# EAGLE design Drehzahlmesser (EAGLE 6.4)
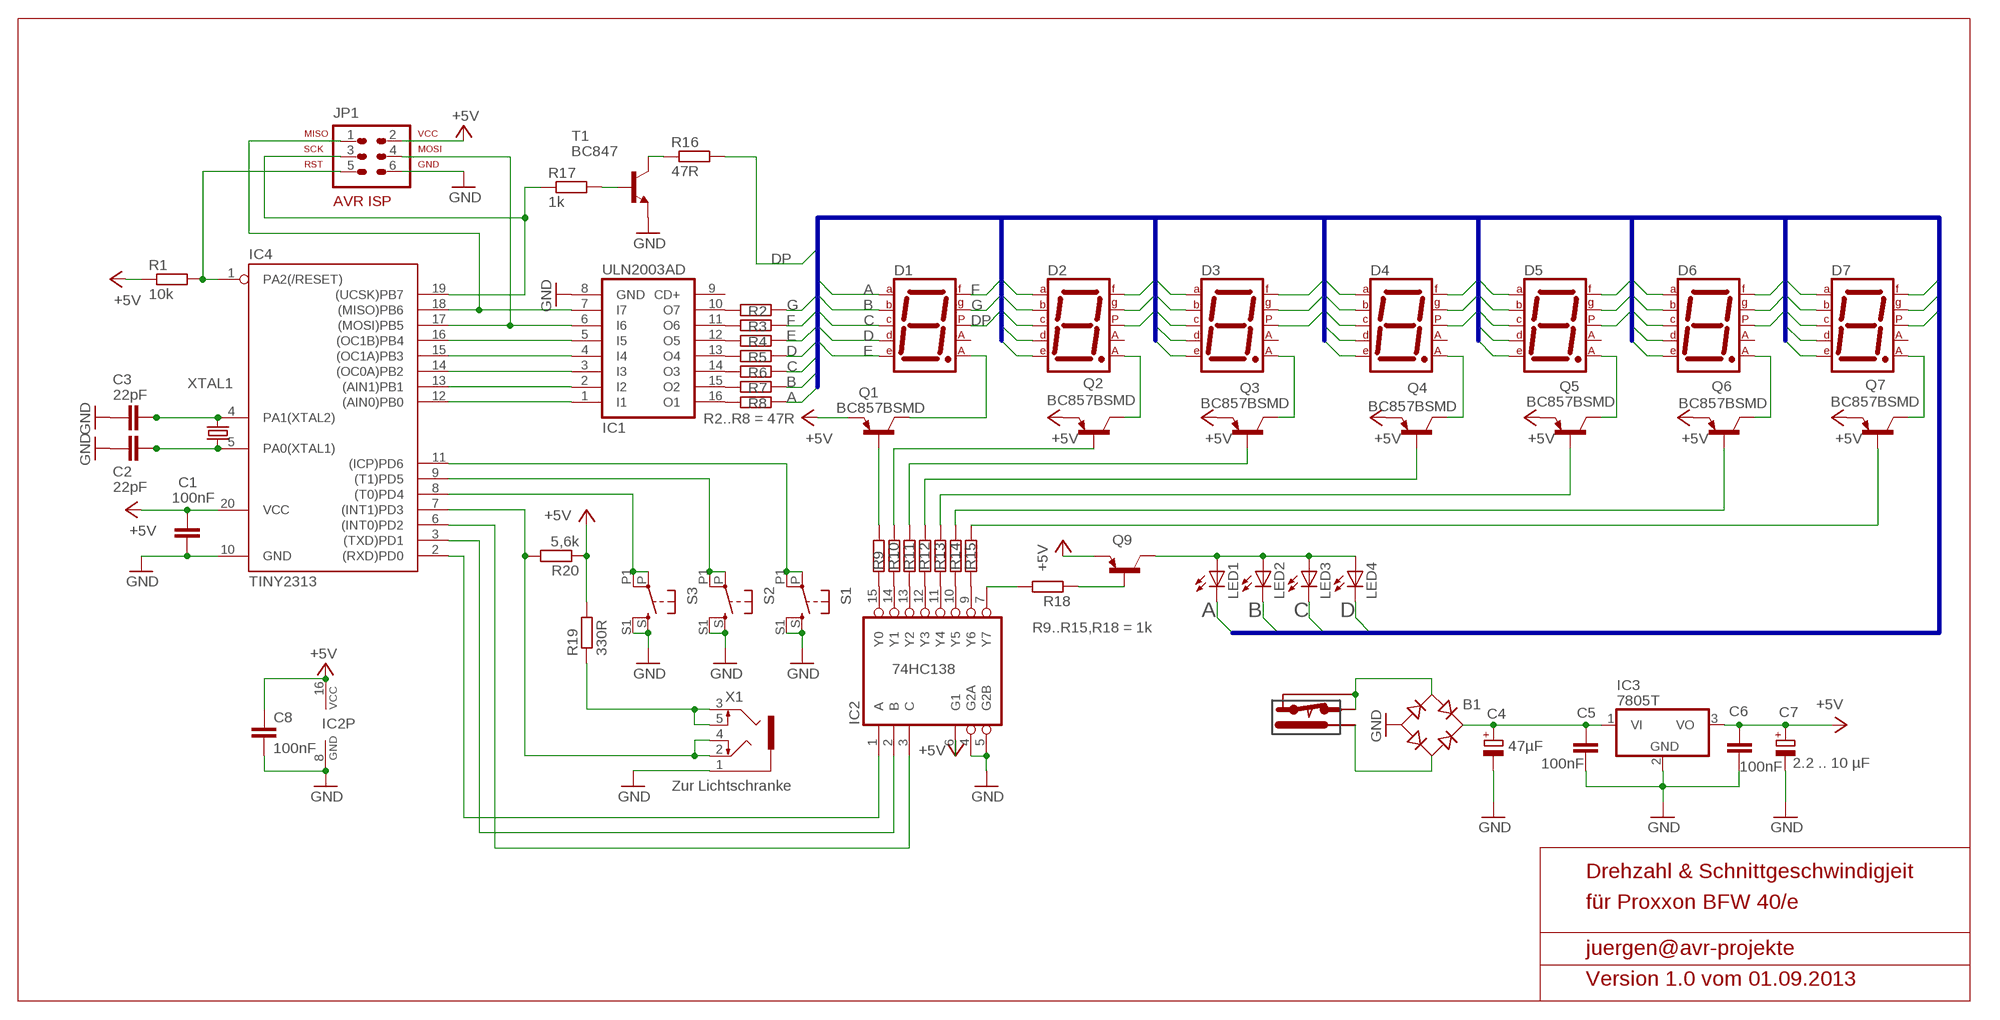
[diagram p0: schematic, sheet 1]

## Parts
B1  RECTIFIER-DIL  [B-DIL]
C1  100nF  C-EUC0805K  [C0805K]
C2  22pF  C-EUC0805  [C0805]
C3  22pF  C-EUC0805  [C0805]
C4  47µF  CPOL-EUE5-10.5  [E5-10,5]
C5  100nF  C-EUC0805K  [C0805K]
C6  100nF  C-EUC0805K  [C0805K]
C7  2.2 .. 10 µF  CPOL-EUE5-5  [E5-5]
C8  100nF  C-EUC0805K  [C0805K]
D1  7SEG-CA  [7SEG-13]
D2  7SEG-CA  [7SEG-13]
D3  7SEG-CA  [7SEG-13]
D4  7SEG-CA  [7SEG-13]
D5  7SEG-CA  [7SEG-13]
D6  7SEG-CA  [7SEG-13]
D7  7SEG-CA  [7SEG-13]
IC1  ULN2003AD  [SO16]
IC2  74HC138  74AC138D  [SO16]
IC3  7805T  [TO220H]
IC4  TINY2313  TINY2313-*S*  [SO20L$]
JP1  AVR-ISP-6VERT  [AVR-ISP-6]
LED1  LED3MM  [LED3MM]
LED2  LED3MM  [LED3MM]
LED3  LED3MM  [LED3MM]
LED4  LED3MM  [LED3MM]
Q1  BC857BSMD  [SOT23-BEC]
Q2  BC857BSMD  [SOT23-BEC]
Q3  BC857BSMD  [SOT23-BEC]
Q4  BC857BSMD  [SOT23-BEC]
Q5  BC857BSMD  [SOT23-BEC]
Q6  BC857BSMD  [SOT23-BEC]
Q7  BC857BSMD  [SOT23-BEC]
Q9  BC857BSMD  [SOT23-BEC]
R1  10k  R-EU_M0805  [M0805]
R2  R-EU_M0805  [M0805]
R3  R-EU_M0805  [M0805]
R4  R-EU_M0805  [M0805]
R5  R-EU_M0805  [M0805]
R6  R-EU_M0805  [M0805]
R7  R-EU_M0805  [M0805]
R8  R-EU_M0805  [M0805]
R9  R-EU_M0805  [M0805]
R10  R-EU_M0805  [M0805]
R11  R-EU_M0805  [M0805]
R12  R-EU_M0805  [M0805]
R13  R-EU_M0805  [M0805]
R14  R-EU_M0805  [M0805]
R15  R-EU_M0805  [M0805]
R16  47R  R-EU_M0805  [M0805]
R17  1k  R-EU_M0805  [M0805]
R18  R-EU_M0805  [M0805]
R19  330R  R-EU_M0805  [M0805]
R20  5,6k  R-EU_M0805  [M0805]
S1  TASTER-SMD-1612-11  [TASTER1612.11]
S2  TASTER-SMD-1612-11  [TASTER1612.11]
S3  TASTER-SMD-1612-11  [TASTER1612.11]
T1  BC847  [SOT23]
U$2  POWERBUCHSE21  [HEBW21]
X1  1503_09  [1503_09]
XTAL1  CRYSTALHC49S  [HC49/S]

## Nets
+5V: C1.1 C6.1 C7.+ C8.1 IC2.6(G1) IC2.16(VCC) IC3.3(VO) IC4.20(VCC) JP1.2 Q1.E Q2.E Q3.E Q4.E Q5.E Q6.E Q7.E Q9.E R1.1 R19.2 R20.1
A: D1.7(A) D2.7(A) D3.7(A) D4.7(A) D5.7(A) D6.7(A) D7.7(A) LED1.K(C) R8.2
B: D1.6(B) D2.6(B) D3.6(B) D4.6(B) D5.6(B) D6.6(B) D7.6(B) LED2.K(C) R7.2
C: D1.4(C) D2.4(C) D3.4(C) D4.4(C) D5.4(C) D6.4(C) D7.4(C) LED3.K(C) R6.2
D: D1.2(D) D2.2(D) D3.2(D) D4.2(D) D5.2(D) D6.2(D) D7.2(D) LED4.K(C) R5.2
DP: D1.5(DP) D2.5(DP) D3.5(DP) D4.5(DP) D5.5(DP) D6.5(DP) D7.5(DP) R16.2
E: D1.1(E) D2.1(E) D3.1(E) D4.1(E) D5.1(E) D6.1(E) D7.1(E) R4.2
F: D1.9(F) D2.9(F) D3.9(F) D4.9(F) D5.9(F) D6.9(F) D7.9(F) R3.2
G: D1.10(G) D2.10(G) D3.10(G) D4.10(G) D5.10(G) D6.10(G) D7.10(G) R2.2
GND: B1.- C1.2 C2.1 C3.1 C4.- C5.2 C6.2 C7.- C8.2 IC1.8(GND) IC2.4(G2A) IC2.5(G2B) IC2.8(GND) IC3.2(GND) IC4.10(GND) JP1.6 S1.S S1.S1 S2.S S2.S1 S3.S S3.S1 T1.2(E) X1.1
LS+: R19.1 X1.3 X1.5
LSOUT: IC4.7((INT1)PD3) R20.2 X1.2 X1.4
N$1: IC4.1(PA2(/RESET)) JP1.5 R1.2
N$2: IC1.1(I1) IC4.12((AIN0)PB0)
N$3: IC1.2(I2) IC4.13((AIN1)PB1)
N$4: IC1.3(I3) IC4.14((OC0A)PB2)
N$5: IC1.4(I4) IC4.15((OC1A)PB3)
N$6: IC1.5(I5) IC4.16((OC1B)PB4)
N$7: IC1.6(I6) IC4.17((MOSI)PB5) JP1.4
N$9: IC2.1(A) IC4.2((RXD)PD0)
N$10: IC2.2(B) IC4.3((TXD)PD1)
N$11: IC2.3(C) IC4.6((INT0)PD2)
N$12: IC1.10(O7) R2.1
N$13: IC1.11(O6) R3.1
N$14: IC1.12(O5) R4.1
N$15: IC1.13(O4) R5.1
N$16: IC1.14(O3) R6.1
N$17: IC1.15(O2) R7.1
N$18: IC1.16(O1) R8.1
N$19: IC2.15(Y0) R9.1
N$20: Q1.B R9.2
N$21: D1.8(CA2) Q1.C
N$22: D2.8(CA2) Q2.C
N$23: Q2.B R10.2
N$24: IC2.14(Y1) R10.1
N$25: IC2.13(Y2) R11.1
N$26: IC2.12(Y3) R12.1
N$27: IC2.11(Y4) R13.1
N$28: IC2.10(Y5) R14.1
N$29: IC2.9(Y6) R15.1
N$30: Q3.B R11.2
N$31: Q4.B R12.2
N$32: Q5.B R13.2
N$33: Q6.B R14.2
N$34: Q7.B R15.2
N$35: D3.8(CA2) Q3.C
N$36: D4.8(CA2) Q4.C
N$37: D5.8(CA2) Q5.C
N$38: D6.8(CA2) Q6.C
N$39: D7.8(CA2) Q7.C
N$40: IC4.19((UCSK)PB7) JP1.3 R17.1
N$41: R17.2 T1.1(B)
N$42: R16.1 T1.3(C)
N$43: C3.2 IC4.4(PA1(XTAL2)) XTAL1.2
N$44: C2.2 IC4.5(PA0(XTAL1)) XTAL1.1
N$46: IC4.11((ICP)PD6) S1.P S1.P1
N$47: IC4.9((T1)PD5) S2.P S2.P1
N$48: IC4.8((T0)PD4) S3.P S3.P1
N$49: IC2.7(Y7) R18.2
N$50: Q9.B R18.1
N$51: LED1.A LED2.A LED3.A LED4.A Q9.C
N$53: B1.AC2 U$2.STIFT
N$55: B1.+ C4.+ C5.1 IC3.1(VI)
N$56: B1.AC1 U$2.MASSE U$2.ÖFFNER
N$57: IC1.7(I7) IC4.18((MISO)PB6) JP1.1
Unconnected: D1.3(CA1) D2.3(CA1) D3.3(CA1) D4.3(CA1) D5.3(CA1) D6.3(CA1) D7.3(CA1) IC1.9(CD+)

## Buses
BUS:A,B,C,D,E,F,G,DP

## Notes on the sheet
- R2..R8 = 47R
- R9..R15,R18 = 1k
- Zur Lichtschranke
- Drehzahl & Schnittgeschwindigjeit
- für Proxxon BFW 40/e
- juergen@avr-projekte
- Version 1.0 vom 01.09.2013

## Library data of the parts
B1 = rectifier:RECTIFIER-: Rectifier
C1-C3 C5 C6 C8 = rcl:C-EU: CAPACITOR, European symbol
C4 C7 = rcl:CPOL-EU: POLARIZED CAPACITOR, European symbol
D1-D7 = special:7SEG-CA: 7-segment DISPLAY single anode, 13 mm
IC1 = uln-udn_x:ULN2003A: DRIVER ARRAY
IC2 = 74xx-eu:74*138: 3-line to 8-line DECODER/DEMULTIPLEXER
IC3 = linear:78*: Positive VOLTAGE REGULATOR Source: http://cache.national.com/ds/LM/LM78L05.pdf http://www.fairchildsemi.com/ds/LM/LM7805.pdf
IC4 = avr-7:TINY2313*: Atmel Tiny2313 2K Flash, 128 bytes EEPROM, 128 bytes RAM
JP1 = avr-7:AVR-ISP-6: AVR ISP-6 Serial Programming Header
LED1-LED4 = led:LED: LED
Q1-Q7 Q9 = transistor-pnp:BC857*: PNP Transistror
R1-R20 = rcl:R-EU_: RESISTOR, European symbol
S1-S3 = 0_jmw:TASTER-SMD-1612-11
T1 = transistor:BC847: NPN TRANSISTOR
U$2 = 0_jmw:POWERBUCHSE21
X1 = con-lumberg:1503_09: Jack connectors according to JISC 6560, 3.5 mm Klinkeneinbaukupplung nach JISC 6560, 3,5 mm, 3-polig/ stereo, abgewinkelte Ausführung, mit 2 Öffnern und Lötaugen, für Leiterplatten Rückseitenmontage Source: http://www.lumberg.com/Produkte/PDFs/1503_09.pdf; OC_FARNELL: 1243244; OC_NEWARK: unknown
XTAL1 = crystal:CRYSTAL: CRYSTAL; OC_FARNELL: 1667008; OC_NEWARK: unknown

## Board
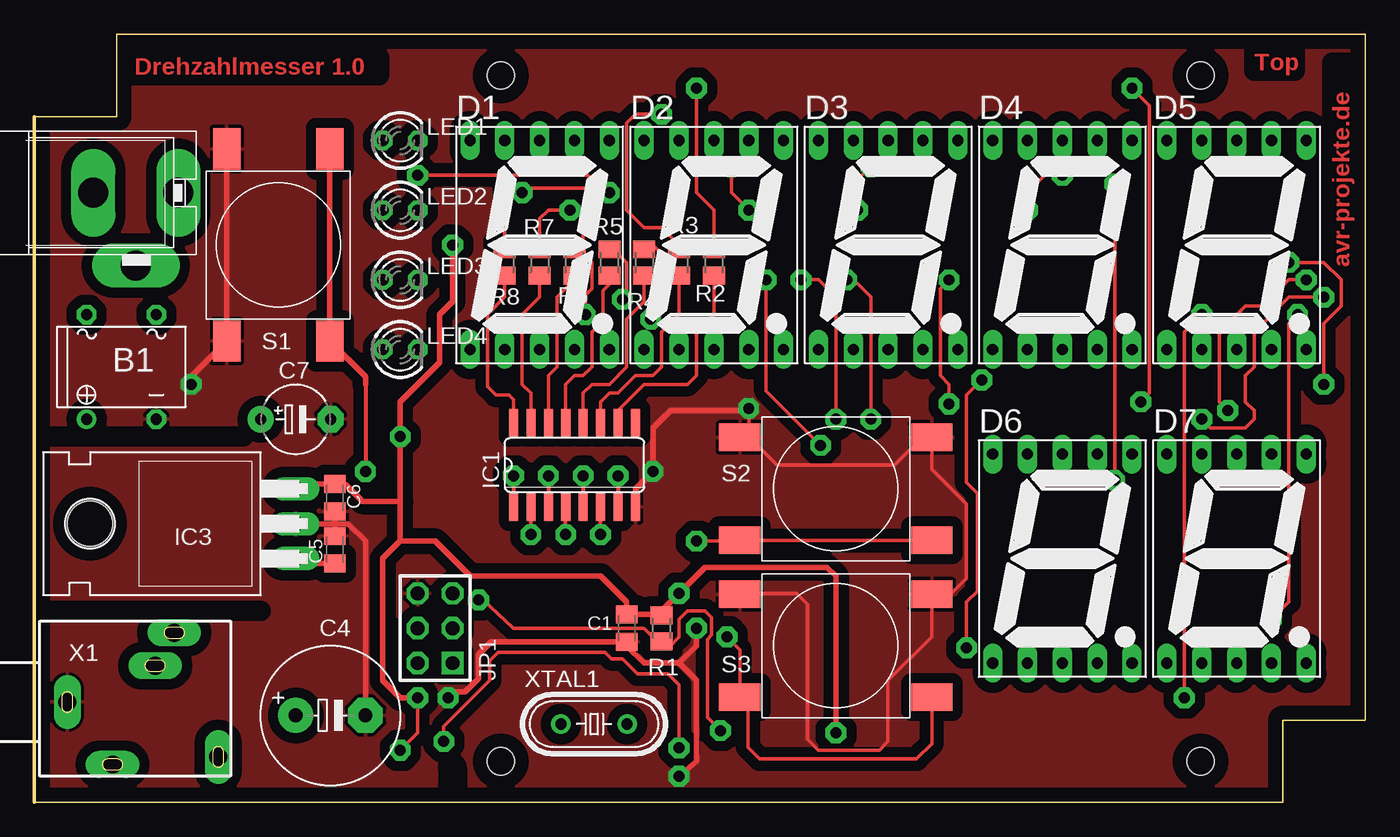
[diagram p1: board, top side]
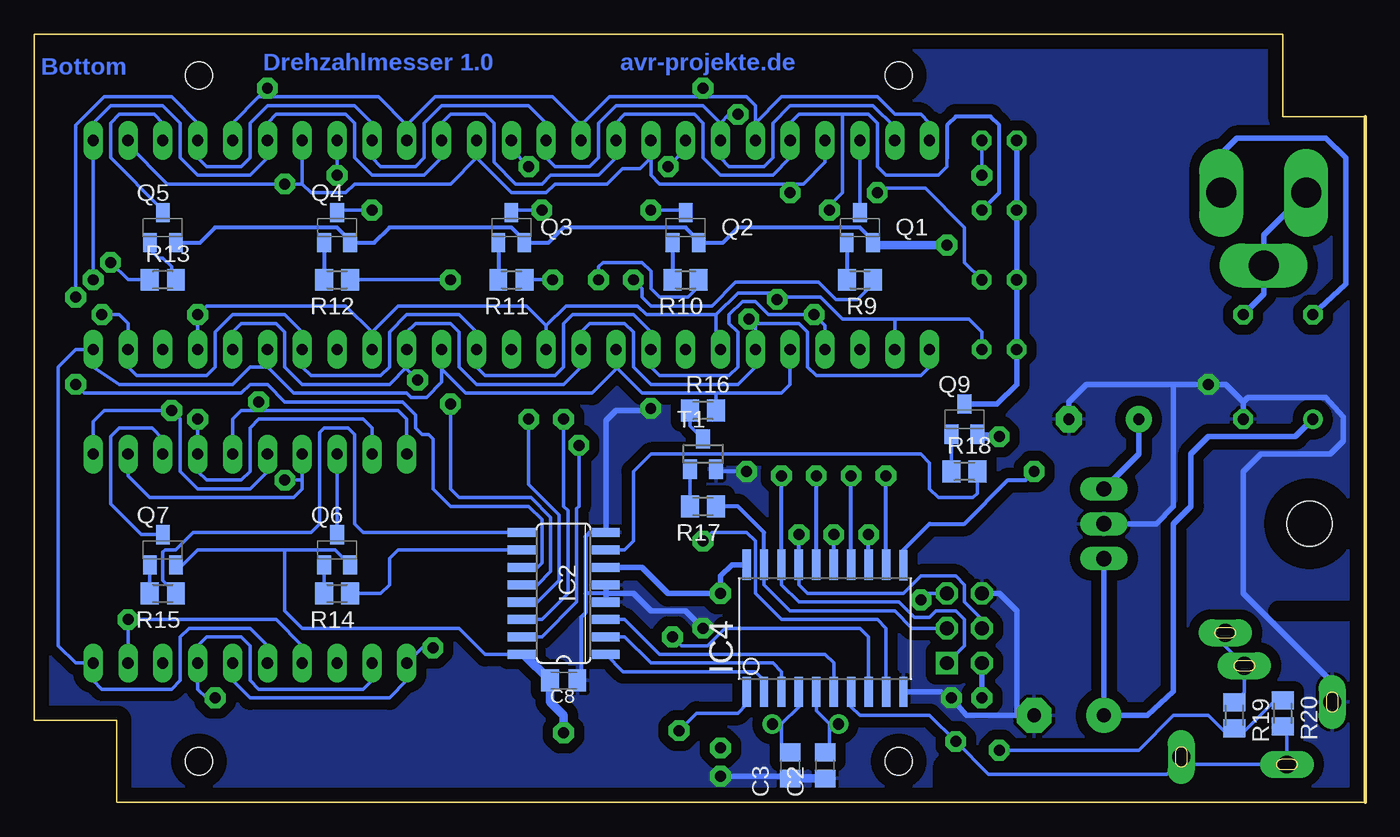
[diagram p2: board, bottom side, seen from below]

Size 97 x 56 mm. Coordinates in mm from the lower left corner, seen from the top.
Outline: 0,50 6,50 6,56 97,56 97,6 91,6 91,0 0,0 0,50
Copper layers (1*16): Top 0.035mm / dielectric 1.5mm / Bottom 0.035mm
Design rules "default *": minimum track width 10mil, minimum drill 24mil, track to track 8mil, track to pad 8mil, pad to pad 8mil, via to via 8mil, smd to smd 8mil, copper to edge 40mil, drill to drill 8mil, minimum pad ring 12mil, minimum via ring 14mil, stop-mask expansion 4mil, vias tented up to drill 0mil, thermal gap 10mil
Holes 2 mm at 34,53 85,53 85,3 34,3
tRestrict: 3 lines
bRestrict: 2 lines

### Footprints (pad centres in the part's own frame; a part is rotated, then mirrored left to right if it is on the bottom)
B-DIL = drill 0.813: + -2.54,-3.81 | drill 0.813 octagon: - 2.54,-3.81; AC1 2.54,3.81; AC2 -2.54,3.81
C0805K = smd 1.3 x 1.6: 1 -1,0; 2 1,0
C0805 = smd 1.3 x 1.5: 1 -0.95,0; 2 0.95,0
E5-10,5 = drill 1.016 pad 2.54: + -2.54,0 | drill 1.016 pad 2.54 octagon: - 2.54,0
E5-5 = drill 0.813 pad 1.905: + -2.54,0 | drill 0.813 pad 1.905 octagon: - 2.54,0
7SEG-13 = drill 0.813 long: 1 -5.08,-7.62; 2 -2.54,-7.62; 3 0,-7.62; 4 2.54,-7.62; 5 5.08,-7.62; 6 5.08,7.62; 7 2.54,7.62; 8 0,7.62; 9 -2.54,7.62; 10 -5.08,7.62
SO16 = smd 0.66 x 2.032: 1 -4.445,-3.073; 2 -3.175,-3.073; 3 -1.905,-3.073; 4 -0.635,-3.073; 5 0.635,-3.073; 6 1.905,-3.073; 7 3.175,-3.073; 8 4.445,-3.073; 9 4.445,3.073; 10 3.175,3.073; 11 1.905,3.073; 12 0.635,3.073; 13 -0.635,3.073; 14 -1.905,3.073; 15 -3.175,3.073; 16 -4.445,3.073
TO220H = drill 1.118 long: 1 -2.54,-10.16; 2 0,-10.16; 3 2.54,-10.16 | hole 3.302: 0,4.826
SO20L$ = smd 0.61 x 2.21: 1 -5.715,-4.636; 2 -4.445,-4.636; 3 -3.175,-4.636; 4 -1.905,-4.636; 5 -0.635,-4.636; 6 0.635,-4.636; 7 1.905,-4.636; 8 3.175,-4.636; 9 4.445,-4.636; 10 5.715,-4.636; 11 5.715,4.61; 12 4.445,4.636; 13 3.175,4.636; 14 1.905,4.636; 15 0.635,4.636; 16 -0.635,4.636; 17 -1.905,4.636; 18 -3.175,4.636; 19 -4.445,4.636; 20 -5.715,4.636
AVR-ISP-6 = drill 1.016 square: 1 -2.54,-1.27 | drill 1.016 octagon: 2 -2.54,1.27; 3 0,-1.27; 4 0,1.27; 5 2.54,-1.27; 6 2.54,1.27
LED3MM = drill 0.813 octagon: A -1.27,0; K 1.27,0
SOT23-BEC = smd 1 x 1.4: B -0.95,-1.1; C 0,1.1; E 0.95,-1.1
M0805 = smd 1.3 x 1.6: 1 -0.95,0; 2 0.95,0
TASTER1612.11 = smd 3 x 2: P -7,3.75; P1 7,3.75; S -7,-3.75; S1 7,-3.75
SOT23 = smd 1 x 1.4: 1 -0.95,-1.1; 2 0.95,-1.1; 3 0,1.1
HEBW21 = drill 2.184 pad 2.54 long: MASSE 0,6.5; STIFT 0,0.3; ÖFFNER -5.3,3.4
1503_09 = drill 1.3 pad 1.676 long: 1 0,-2.1; 2 -4.55,-5.4; 3 5.05,-9.9; 4 -4,-13.1; 5 2.65,-8.5
HC49/S = drill 0.813: 1 -2.413,0; 2 2.413,0

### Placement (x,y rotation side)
B1  6.35,31.75 0 top
C1  43.18,12.7 270 top
C2  39.37,2.7 90 bottom
C3  41.91,2.7 90 bottom
C4  21.59,6.35 0 top
C5  21.91,18.41 90 top
C6  21.91,22.23 270 top
C7  19.05,27.94 0 top
C8  58.42,8.89 0 bottom
D1  36.83,40.64 0 top
D2  49.53,40.64 0 top
D3  62.23,40.64 0 top
D4  74.93,40.64 0 top
D5  87.63,40.64 0 top
D6  74.93,17.78 0 top
D7  87.63,17.78 0 top
IC1  39.37,24.61 0 top
IC2  58.42,15.24 90 bottom
IC3  8.89,20.32 90 top
IC4  39.37,12.7 0 bottom
JP1  29.21,12.7 90 top
LED1  26.67,48.26 0 top
LED2  26.67,43.18 0 top
LED3  26.67,38.1 0 top
LED4  26.67,33.02 0 top
Q1  36.83,41.91 0 bottom
Q2  49.53,41.91 0 bottom
Q3  62.23,41.91 0 bottom
Q4  74.93,41.91 0 bottom
Q5  87.63,41.91 0 bottom
Q6  74.93,18.41 0 bottom
Q7  87.63,18.41 0 bottom
Q9  29.21,27.94 0 bottom
R1  45.72,12.7 270 top
R2  49.53,39.37 90 top
R3  46.99,39.37 90 top
R4  44.45,39.37 90 top
R5  41.91,39.37 90 top
R6  39.37,39.37 90 top
R7  36.83,39.37 90 top
R8  34.29,39.37 90 top
R9  36.83,38.1 180 bottom
R10  49.53,38.1 180 bottom
R11  62.23,38.1 180 bottom
R12  74.93,38.1 180 bottom
R13  87.63,38.1 0 bottom
R14  74.93,15.24 180 bottom
R15  87.63,15.24 180 bottom
R16  48.26,28.57 0 bottom
R17  48.26,21.59 180 bottom
R18  29.21,24.13 0 bottom
R19  9.53,6.35 270 bottom
R20  6,6.5 270 bottom
S1  17.78,40.64 270 top
S2  58.42,22.86 180 top
S3  58.42,11.43 180 top
T1  48.26,25.4 0 bottom
U$2  10.79,44.45 90 top
X1  0.3,7.32 90 top
XTAL1  40.8,5.71 0 top

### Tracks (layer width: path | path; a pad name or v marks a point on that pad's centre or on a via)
+5V  (via drill 0.8, 0.8 pad 0.81)
  Top 0.254: v26.67,3.81 27.94,5.08 v27.94,7.62
  Top 0.406: 45.67,13.7 C1.1 43.18,14.61 41.27,16.51 31.75,16.51 29.21,19.05 26.67,19.05 | 45.72,13.97 v46.99,15.24 48.9,17.14 57.78,17.14 58.42,16.51 v58.42,5.08 | 26.67,19.05 25.4,17.78 25.4,8.89 26.67,7.62 v27.94,7.62 | v30.48,40.64 30.48,36.51 29.53,35.56 29.53,32.07 26.67,29.21 v26.67,26.67 26.67,21.91 | 26.67,19.05 26.67,21.91 | 26.67,21.91 26.62,21.95 23.92,21.95 22.7,23.18 C6.1 19.41,23.23 IC3.3
  Top 0.61: 45.67,13.7 R1.1 45.72,13.97
  Bottom 0.254: Q7.E 86.19,17.32 85.09,18.41 78.74,18.41 | 78.74,18.41 75.08,18.41 Q6.E | IC2.16 64.14,10.79 66.04,12.7 77.47,12.7 78.74,13.97 78.74,18.41 | v26.67,3.81 16.51,3.81 13.97,6.35 11.43,6.35 10.16,5.08 | 9.85,5.08 8.92,5.08 6.5,7.5 6.05,7.5 R20.1
  Bottom 0.305: Q1.E 35.88,40.96 36.83,41.91 45.72,41.91 46.82,40.81 Q2.E 48.58,40.96 49.53,41.91 58.42,41.91 59.52,40.81 Q3.E 61.28,40.96 62.23,41.91 71.12,41.91 72.22,40.81 Q4.E 73.98,40.96 74.93,41.91 83.82,41.91 84.92,40.81 Q5.E
  Bottom 0.406: IC4.20 46.16,17.34 46.99,16.51 v46.99,15.24 50.8,15.24 52.7,17.14 IC2.6 | v27.94,7.62 JP1.2 | 10.16,5.08 9.85,5.08 R19.2 | C7.+ 16.51,25.4 IC3.3
  Bottom 0.61: v58.42,5.08 58.42,6.35 59.42,7.35 C8.1 61.33,10.79 IC2.16 | v26.67,26.67 28.09,26.67 Q9.E | v30.48,40.64 35.71,40.64 Q1.E
A  (via drill 0.8)
  Top 0.254: R8.2 34.29,45.72 | v78.74,23.5 v78.74,45.09 | 34.29,45.72 40.32,45.72 41.59,44.45 v41.91,44.45 | 34.29,45.72 v27.94,45.72
  Bottom 0.254: D5.7 90.17,47.94 87.31,45.09 v78.74,45.09 77.47,45.09 | 77.47,23.5 77.47,22.86 78.11,22.23 88.58,22.23 90.17,23.81 D7.7 | D6.7 77.47,23.5 | 77.47,23.5 v78.74,23.5 | D1.7 39.37,46.67 40.96,45.09 41.91,45.09 | v27.94,45.72 LED1.K | D2.7 52.07,46.99 | 52.07,46.99 52.07,45.72 51.44,45.09 41.91,45.09 | 64.77,46.99 62.23,44.45 59.69,44.45 59.05,45.09 55.24,45.09 54.13,46.2 52.86,46.2 52.07,46.99 | D3.7 64.77,46.99 | 64.77,46.99 66.67,45.09 73.66,45.09 74.3,44.45 76.83,44.45 77.47,45.09 | 77.47,45.09 D4.7 | v41.91,44.45 41.91,45.09
B  (via drill 0.8, 0.8 pad 0.81)
  Top 0.254: v87,28.57 86.36,29.21 86.36,34.29 88.27,36.2 89.53,36.2 91.44,38.1 v92.71,38.1 | R7.2 36.83,42.55 37.47,43.18 v39.05,43.18
  Bottom 0.254: D6.6 80.01,24.13 81.28,22.86 85.09,22.86 86.36,24.13 86.36,27.94 v87,28.57 91.92,28.57 92.71,27.78 D7.6 | v92.71,38.1 D5.6 92.71,49.53 91.44,50.8 87.63,50.8 86.36,49.53 86.36,46.99 85.09,45.72 81.28,45.72 80.01,46.99 D4.6 80.01,49.53 79.38,50.16 74.3,50.16 73.66,49.53 73.66,46.99 72.39,45.72 68.58,45.72 67.31,46.99 D3.6 67.31,49.53 66.67,50.16 64.14,50.16 63.5,49.53 63.5,46.67 61.91,45.09 60.01,45.09 59.37,45.72 55.88,45.72 54.61,46.99 D2.6 54.61,49.53 53.98,50.16 48.9,50.16 48.26,49.53 48.26,46.99 46.99,45.72 43.18,45.72 41.91,46.99 D1.6 41.91,49.53 41.27,50.16 38.1,50.16 | 38.1,50.16 36.2,50.16 35.56,49.53 35.56,46.35 34.92,45.72 31.11,45.72 30.48,46.35 30.48,46.99 30.48,47.62 | v39.05,43.18 39.05,43.5 38.1,44.45 38.1,50.16
  Bottom 0.305: LED2.K 26.67,44.45 26.67,49.37 27.3,50.01 29.84,50.01 30.48,49.37 30.48,46.99
C  (via drill 0.8, 0.8 pad 0.81)
  Top 0.254: v90.17,13.34 91.44,14.61 91.44,34.92 v92.08,35.56 | R6.2 39.05,40.32 | R6.2 39.69,40.32 40.64,39.37 40.64,37.47 40.16,36.99 v40.16,35.56 | v35.56,44.45 35.56,44.77 40.16,44.77 40.64,44.29 40.64,42.23 40.01,41.59 40.01,40.95 R6.2
  Bottom 0.254: D1.4 39.37,34.77 v40.16,35.56 43.5,35.56 44.45,36.51 45.4,36.51 46.35,35.56 46.35,34.92 45.72,34.29 45.72,31.75 46.35,31.11 51.44,31.11 52.07,31.75 D2.4 52.07,34.29 53.34,35.56 57.78,35.56 58.42,34.92 58.42,31.75 59.05,31.11 64.14,31.11 64.77,31.75 D3.4 64.77,34.29 66.04,35.56 69.85,35.56 71.12,34.29 71.12,31.75 71.75,31.11 76.83,31.11 77.47,31.75 D4.4 77.47,34.29 78.74,35.56 82.55,35.56 83.82,34.29 83.82,31.75 84.45,31.11 89.53,31.11 90.17,31.75 D5.4 90.17,34.92 90.81,35.56 v92.08,35.56 | D6.4 77.47,11.43 79.38,13.34 v90.17,13.34 D7.4 90.17,11.43 | LED3.K 29.21,39.37 29.21,41.91 32.07,44.77 35.56,44.77 v35.56,44.45
D  (via drill 0.8 pad 0.81)
  Top 0.254: v85.09,35.56 83.82,34.29 v83.82,7.62 | 41.59,40.32 R5.2 42.23,40.32 43.18,39.37 43.18,36.99 v42.86,36.67
  Bottom 0.254: D6.2 72.39,8.89 73.03,8.26 80.64,8.26 81.28,8.89 81.28,11.43 81.92,12.06 84.45,12.06 85.09,11.43 D7.2 85.09,8.26 84.45,7.62 v83.82,7.62 | D5.2 v85.09,35.56 84.45,36.2 74.3,36.2 72.39,34.29 | 47.31,35.56 52.39,35.56 53.02,36.2 58.26,36.2 59.69,34.77 | D2.2 46.99,33.66 47.31,33.97 47.31,35.56 | 47.31,35.56 45.72,37.15 43.34,37.15 v42.86,36.67 42.7,36.83 39.69,36.83 38.1,35.24 34.29,35.24 | 34.29,35.24 28.89,35.24 27.94,34.29 LED4.K | D1.2 34.29,35.24 | 59.69,34.77 61.12,36.2 70.48,36.2 72.39,34.29 | 72.39,34.29 D4.2 | 59.69,34.77 D3.2
DP
  Bottom 0.254: D6.5 80.01,11.43 81.28,12.7 85.72,12.7 86.36,12.06 86.36,8.89 87,8.26 92.08,8.26 92.71,8.89 D7.5 93.98,10.16 95.25,11.43 95.25,31.75 93.98,33.02 D5.5 92.71,31.75 90.81,30.48 82.55,30.48 81.28,31.75 80.01,31.75 | 41.91,31.75 D1.5 41.91,30.48 42.55,29.84 47.31,29.84 | 80.01,31.75 78.11,29.84 69.85,29.84 69.53,29.53 68.42,29.53 67.31,30.64 67.31,31.59 | 80.01,31.75 D4.5 | 46.99,29.21 46.99,28.57 R16.2 47.31,29.84 | 47.31,29.84 52.7,29.84 54.61,31.75 D2.5 54.61,31.59 56.36,29.84 65.56,29.84 67.31,31.59 | 67.31,31.59 D3.5
E  (via drill 0.8 pad 0.41, 0.8 pad 0.81)
  Top 0.254: 44.13,40.32 R4.2 44.77,40.64 45.09,40.64 45.72,40.01 45.72,36.04 v44.93,35.24 | v67.94,11.27 67.94,14.61 68.74,15.4 68.74,22.54 67.94,23.34 67.94,29.69 v69.06,30.8
  Bottom 0.254: D6.1 69.85,8.89 71.12,7.62 81.28,7.62 82.55,8.89 D7.1 | D1.1 31.75,31.75 32.38,31.11 40.01,31.11 40.64,31.75 40.64,34.29 41.27,34.92 44.45,34.92 | 44.45,34.92 D2.1 44.45,31.75 45.72,30.48 52.07,30.48 53.34,31.75 53.34,34.29 53.98,34.92 56.52,34.92 57.15,34.29 D3.1 57.15,31.75 58.42,30.48 64.77,30.48 66.04,31.75 66.04,34.29 66.67,34.92 69.22,34.92 69.85,34.29 D4.1 69.85,31.75 | 69.85,31.75 71.12,30.48 77.47,30.48 78.74,31.75 78.74,34.29 79.38,34.92 81.92,34.92 82.55,34.29 D5.1 | 44.45,34.92 v44.93,35.24 | D6.1 69.85,11.43 | v67.94,11.27 68.74,11.27 D6.1 | 69.85,31.75 69.85,31.59 v69.06,30.8
F  (via drill 0.8 pad 0.81)
  Top 0.254: v85.09,27.94 85.72,27.3 88.27,27.3 88.9,27.94 88.9,28.57 88.27,29.21 88.27,31.11 88.9,31.75 88.9,34.29 91.44,36.83 v93.98,36.83 | R3.2 46.99,40.64 45.72,41.91 44.45,41.91 43.18,43.18 43.18,49.53 43.81,50.16 v45.72,50.16
  Bottom 0.254: D1.9 34.29,49.21 35.88,50.8 41.91,50.8 43.18,49.53 43.18,46.99 43.81,46.35 46.35,46.35 46.99,46.99 D2.9 46.99,49.53 | 46.99,49.53 48.26,50.8 54.61,50.8 55.88,49.53 55.88,46.99 56.52,46.35 59.05,46.35 59.69,46.99 D3.9 59.69,49.53 60.96,50.8 67.31,50.8 68.58,49.53 68.58,46.99 69.22,46.35 71.75,46.35 72.39,46.99 D4.9 72.39,49.53 73.66,50.8 80.01,50.8 81.28,49.53 81.28,46.99 81.92,46.35 84.45,46.35 85.09,46.99 D5.9 85.09,49.53 87,51.44 91.92,51.44 93.98,49.37 v93.98,36.83 | D6.9 72.39,27.3 73.03,27.94 80.64,27.94 81.28,27.3 81.28,24.13 81.92,23.5 84.45,23.5 85.09,24.13 D7.9 v85.09,27.94 | v45.72,50.16 46.35,50.16 46.99,49.53
G  (via drill 0.8 pad 0.81)
  Top 0.254: v80.64,29.21 81.28,29.84 81.28,50.8 v80.01,52.07 | R2.2 49.53,43.18 48.26,44.45 v48.26,52.07
  Bottom 0.254: D1.10 31.75,49.53 32.38,50.16 34.29,50.16 35.56,51.44 42.55,51.44 44.45,49.53 | 80.01,51.44 80.64,51.44 82.55,49.53 D5.10 | D6.10 69.85,27.94 70.48,28.57 80.64,28.57 | 80.64,28.57 81.92,28.57 82.55,27.94 D7.10 | v80.64,29.21 80.64,28.57 | v48.26,52.07 48.26,51.44 | v80.01,52.07 80.01,51.44 | 44.45,49.53 D2.10 | 48.26,51.44 45.09,51.44 44.45,50.8 44.45,49.53 | 57.15,49.37 55.09,51.44 48.26,51.44 | D3.10 57.15,49.37 | 57.15,49.37 59.21,51.44 67.79,51.44 69.85,49.37 | 69.85,49.37 D4.10 | 80.01,51.44 71.91,51.44 69.85,49.37
GND  (via drill 0.8, 0.8 pad 0.81)
  Top 0.254: v52.07,28.73 52.07,27.26 51.77,26.96 | 51.77,26.96 S2.S1 | 50.74,15.18 S3.S1 51.48,15.24 55.56,15.24 56.36,14.45 56.36,4.6 57.15,3.81 61.59,3.81 62.23,4.45 62.23,8.89 65.42,12.08 S3.S 65.48,15.24 66.83,15.24 67.94,16.35 67.94,21.75 65.42,24.27 S2.S 65.36,26.67 64.77,26.67 62.71,24.61 54.13,24.61 51.77,26.96
  Top 0.406: C1.2 33.29,11.7 32.38,10.79 32.38,9.05 31.4,8.06 30.61,8.06 v30.16,7.62 | 43.18,11.43 44.45,10.16 46.99,10.16 | 46.99,10.16 48.26,11.43 v48.26,12.7 | 46.99,10.16 48.26,8.89 48.26,3.02 v46.99,1.91 | 52.07,28.57 46.35,28.57 45.09,27.3 v45.09,24.13 43.81,22.86 IC1.8 | C4.- 24.13,19.05 22.86,20.32 21.91,20.32 | C5.2 21.91,20.32 | 21.91,20.32 C6.2 | IC3.2 21.91,20.32 | v11.43,30.48 11.43,31.04 S1.S1 S1.S
  Top 0.61: C1.2 43.18,11.43
  Bottom 0.305: v45.09,24.13 47.14,24.13 T1.2 | IC2.8 56.52,19.68 56.83,19.37 56.83,15.24 | 56.83,15.24 56.83,13.81 57.15,13.49 57.15,9.48 | 55.35,15.24 56.83,15.24
  Bottom 0.406: IC2.4 55.35,15.24 | 55.35,15.24 IC2.5 55.35,15.34 55.24,15.24 | 55.24,15.24 53.34,15.24 52.07,13.97 49.53,13.97 v48.26,12.7 | 55.24,15.24 55.35,15.24 | C8.2 57.15,8.89 56.99,9.05 | v46.99,1.91 42.55,1.91 42.23,1.59 42.23,1.58 42.23,1.27 | IC2.8 55.35,27.84 54.61,28.57 52.07,28.57 | JP1.6 26.67,15.24 25.4,13.97 25.4,6.35 | C4.- 25.4,6.35 | 25.4,6.35 29.05,6.35 v30.16,7.62 30.92,8.06 IC4.10 | B1.- 8.89,29.21 | 8.89,29.21 10.16,30.48 v11.43,30.48 13.97,30.48 | 13.97,30.48 20.32,30.48 21.59,29.21 C7.- | 57.1,9.21 C8.2 | C8.2 56.99,9.32 57.15,9.48 | 8.89,29.21 8.57,29.53 2.86,29.53 1.59,28.1 1.59,26.35 2.54,25.4 7.62,25.4 8.89,24.13 8.89,15.24 2.4,8.75 X1.1 | 13.97,30.48 13.97,21.59 15.24,20.32 IC3.2
  Bottom 0.61: C3.1 C2.1
  pour Bottom (isolate 0.75): -1.27,-1.27 97.79,-1.27 97.79,57.15 -1.27,57.15
  pour Top (isolate 0.75): -1.27,57.15 -1.27,-1.27 97.79,-1.27 97.79,57.15
LS+
  Bottom 0.254: X1.3 10.2,11.37 X1.5 8.8,8.02 R19.1
LSOUT  (via drill 0.8)
  Top 0.254: v29.84,4.45 29.84,5.56 33.18,8.89 33.18,10.32 33.81,10.95 41.59,10.95 42.07,10.48 42.86,10.48 43.97,9.37 46.2,9.37 46.99,8.57 v46.99,3.97
  Bottom 0.254: IC4.7 37.47,6.99 36.83,6.35 31.75,6.35 v29.84,4.45 27.45,2.05 27.44,2.06 14.45,2.06 13.4,3.11 X1.4 12.85,2.77 X1.2 5.7,5.55 R20.2
N$1  (via drill 0.8 pad 0.81)
  Top 0.254: v32.38,14.76 32.7,14.76 34.92,12.7 44.45,12.7 45.4,11.75 R1.2 46.04,11.43 46.35,11.43 46.99,12.06 46.99,13.34 47.62,13.97 48.9,13.97 49.37,13.49 49.37,12.22 49.05,11.91 49.05,6.19 v50.01,5.24
  Bottom 0.254: v50.01,5.24 48.74,6.51 45.72,6.51 45.09,7.14 45.05,7.14 IC4.1 | v32.38,14.76 31.91,15.24 JP1.5
N$2  (via drill 0.8 pad 0.81)
  Top 0.305: v34.92,23.81 IC1.1
  Bottom 0.305: IC4.12 v34.92,23.81
N$3  (via drill 0.8 pad 0.81)
  Top 0.305: v36.2,19.53 IC1.2
  Bottom 0.305: IC4.13 v36.2,19.53
N$4  (via drill 0.8 pad 0.81)
  Top 0.305: v37.47,23.81 IC1.3
  Bottom 0.305: IC4.14 v37.47,23.81
N$5  (via drill 0.8 pad 0.81)
  Top 0.305: v38.73,19.53 IC1.4
  Bottom 0.305: IC4.15 v38.73,19.53
N$6  (via drill 0.8 pad 0.81)
  Top 0.305: v40.01,23.81 IC1.5
  Bottom 0.305: IC4.16 v40.01,23.81
N$7  (via drill 0.8 pad 0.81)
  Top 0.305: v41.27,19.53 IC1.6
  Bottom 0.254: JP1.4 27.94,13.34 29.21,14.61 29.21,15.88 29.84,16.51 32.38,16.51 33.66,15.24 40.64,15.24 41.27,15.88 IC4.17
  Bottom 0.305: IC4.17 v41.27,19.53
N$9
  Bottom 0.254: IC4.2 43.81,8.89 44.45,9.53 54.08,9.53 IC2.1
N$10
  Bottom 0.254: IC4.3 42.55,9.53 43.18,10.16 52.07,10.16 53.98,12.06 IC2.2
N$11
  Bottom 0.254: IC2.3 53.98,13.34 51.44,10.79 39.37,10.79 38.73,10.16 IC4.6
N$12
  Top 0.254: IC1.10 42.55,28.57 44.45,30.48 47.62,30.48 48.26,31.11 48.26,34.29 49.53,35.56 R2.1
N$13
  Top 0.254: IC1.11 41.27,29.21 41.91,29.84 42.55,29.84 43.81,31.11 45.09,31.11 45.72,31.75 45.72,34.29 46.99,35.56 R3.1
N$14
  Top 0.254: 44.45,38.1 R4.1 44.45,36.51 43.18,35.24 43.18,31.75 41.91,30.48 40.64,30.48 40.01,29.84 IC1.12
N$15
  Top 0.254: IC1.13 38.73,30.48 39.37,31.11 40.01,31.11 40.64,31.75 40.64,34.29 41.43,35.08 41.43,37.31 41.91,37.78 R5.1
N$16
  Top 0.254: R6.1 39.37,38.1 38.1,36.83 38.1,31.75 37.47,31.11 IC1.14
N$17
  Top 0.254: R7.1 36.83,36.83 35.56,35.56 35.56,30.48 36.2,29.84 IC1.15
N$18
  Top 0.254: R8.1 34.29,36.83 33.02,35.56 33.02,30.32 33.66,29.69 34.61,29.69 34.92,29.37 IC1.16
N$19  (via drill 0.8, 0.8 pad 0.81)
  Top 0.254: v53.34,38.1 53.34,30 v57.31,26.04
  Bottom 0.254: R9.1 35.88,37.78 36.99,36.67 38.58,36.67 39.85,37.94 45.88,37.94 47.62,36.2 52.07,36.2 52.7,36.83 52.7,37.47 v53.34,38.1 | v57.31,26.04 57.31,21.59 57.47,21.43 57.47,14.61 60.01,12.06 IC2.15
N$20
  Bottom 0.305: Q1.B R9.2
N$21
  Bottom 0.254: D1.8 Q1.C
N$22  (via drill 0.8 pad 0.81)
  Top 0.254: v50.8,46.35 50.8,44.45 v52.07,43.18
  Bottom 0.254: D2.8 49.53,47.62 v50.8,46.35 | v52.07,43.18 49.7,43.18 Q2.C
N$23
  Bottom 0.305: Q2.B R10.2
N$24  (via drill 0.8, 0.8 pad 0.81)
  Top 0.254: v55.88,38.1 57.15,38.1 58.42,36.83 v58.42,27.94
  Bottom 0.254: R10.1 48.58,37.94 48.58,37.62 49.37,36.83 51.44,36.83 52.07,37.47 52.07,38.73 52.7,39.37 55.56,39.37 55.88,39.05 v55.88,38.1 | v58.42,27.94 58.42,21.59 58.1,21.27 58.1,15.24 60.01,13.34 IC2.14
N$25  (via drill 0.8 pad 0.81)
  Top 0.254: v60.96,27.94 60.96,36.83 59.69,38.1 v59.21,38.1
  Bottom 0.254: IC2.13 60.33,14.61 58.74,16.19 58.74,20.95 60.96,23.18 v60.96,27.94 | v59.21,38.1 R11.1
N$26  (via drill 0.8 pad 0.81)
  Top 0.254: v66.67,29.05 66.67,30.48 66.04,31.11 66.04,37.47 v66.67,38.1
  Bottom 0.254: IC2.12 60.33,15.88 59.37,16.83 59.37,20.8 60.8,22.23 66.04,22.23 66.67,22.86 v66.67,29.05 | v66.67,38.1 R12.1
N$27  (via drill 0.8 pad 0.41, 0.8 pad 0.81)
  Top 0.254: v93.98,30.48 93.98,34.92 95.25,36.2 95.25,38.1 93.98,39.37 v91.44,39.37
  Bottom 0.254: IC2.11 60.33,17.14 60.01,17.46 60.01,20.64 60.96,21.59 66.67,21.59 67.94,22.86 67.94,26.51 68.26,26.83 68.74,26.83 69.22,27.3 69.22,28.26 70.17,29.21 78.74,29.21 80.01,30.48 81.28,30.48 81.92,29.84 93.34,29.84 v93.98,30.48 | v91.44,39.37 90.17,38.1 R13.1
N$28
  Bottom 0.254: IC2.10 70.48,18.41 71.12,17.78 71.12,15.88 71.75,15.24 R14.1
N$29
  Bottom 0.254: IC2.9 73.03,19.68 73.66,20.32 73.66,26.83 74.14,27.3 75.88,27.3 76.2,26.99 76.2,20.32 76.83,19.68 85.41,19.68 86.68,18.41 87.47,18.41 87.63,18.26 87.63,16.19 R15.1
N$30
  Bottom 0.305: Q3.B R11.2
N$31
  Bottom 0.305: Q4.B R12.2
N$32
  Bottom 0.254: Q5.B 88.58,40.32 87.95,39.69 87.63,39.69 87,39.05 87,38.41 R13.2
N$33
  Bottom 0.254: Q6.B R14.2
N$34
  Bottom 0.254: Q7.B R15.2
N$35  (via drill 0.8 pad 0.41)
  Top 0.254: v60.96,46.35 60.01,45.4 v60.01,43.18
  Bottom 0.254: D3.8 62.23,47.62 v60.96,46.35 | v60.01,43.18 62.06,43.18 Q3.C
N$36  (via drill 0.8 pad 0.41)
  Top 0.254: v74.93,45.72 73.66,45.72 72.39,44.45 v72.39,43.18
  Bottom 0.254: D4.8 v74.93,45.72 | v72.39,43.18 74.76,43.18 Q4.C
N$37
  Bottom 0.254: Q5.C 87.63,43.18 91.44,46.99 91.44,49.53 90.81,50.16 88.27,50.16 87.63,49.53 D5.8
N$38
  Bottom 0.254: Q6.C D6.8
N$39
  Bottom 0.254: D7.8 87.63,26.51 88.42,27.3 90.81,27.3 91.44,26.67 91.44,21.75 89.22,19.53 87.64,19.53 Q7.C
N$40
  Bottom 0.254: JP1.3 33.02,12.7 34.29,13.97 41.91,13.97 43.81,15.88 IC4.19
  Bottom 0.305: IC4.19 43.81,19.68 45.72,21.59 R17.1
N$41
  Bottom 0.254: R17.2 T1.1
N$42
  Bottom 0.254: R16.1 49.21,27.45 T1.3
N$43
  Bottom 0.254: IC4.4 41.27,6.99 42.55,5.71 | 42.55,5.71 42.55,4.28 C3.2 | XTAL1.2 42.55,5.71
N$44
  Bottom 0.254: IC4.5 40.01,6.67 39.05,5.71 | 39.05,5.71 39.05,3.97 C2.2 | XTAL1.1 39.05,5.71
N$46  (via drill 0.8)
  Top 0.305: 24.13,30.48 v24.13,24.13
  Top 0.406: 24.13,30.48 24.13,31.04 S1.P1 S1.P
  Bottom 0.305: IC4.11 33.66,18.41 31.75,20.32 29.21,20.32 26.04,23.5 24.77,23.5 v24.13,24.13
N$47  (via drill 0.8 pad 0.81)
  Top 0.254: v48.26,19.05 51.36,19.05 S2.P1 S2.P
  Bottom 0.254: v48.26,19.05 47.62,19.68 45.09,19.68 44.45,19.05 44.45,15.24 42.55,13.34 35.56,13.34 34.92,12.7 IC4.9
N$48  (via drill 0.8)
  Top 0.254: v50.48,12.06 51.42,11.13 S3.P1 52.01,7.68 52.01,4.03 52.86,3.17 64.29,3.17 65.41,4.29 65.41,7.67 S3.P 65.48,7.62 66.04,7.62
  Bottom 0.254: IC4.8 36.2,12.06 36.83,12.7 46.67,12.7 47.94,11.43 49.85,11.43 v50.48,12.06
N$49
  Bottom 0.254: R18.2 28.26,22.54 28.57,22.23 31.11,22.23 31.75,22.86 31.75,24.77 32.38,25.4 52.07,25.4 53.34,24.13 53.34,19.05 53.98,18.41 IC2.7
N$50
  Bottom 0.254: R18.1 Q9.B
N$51
  Bottom 0.406: Q9.C 26.84,29.04 25.4,30.48 LED4.A LED3.A LED2.A LED1.A
N$53
  Bottom 0.406: B1.AC2 1.43,37.78 1.43,46.99 2.86,48.42 9.37,48.42 10.48,47.31 | 10.48,44.47 U$2.STIFT
  Bottom 0.61: 10.48,47.31 10.48,44.47
N$55
  Top 0.406: C5.1 19.41,17.41 IC3.1
  Bottom 0.406: IC3.1 C4.+ 15.88,6.35 13.97,8.1 13.97,20.32 12.7,21.59 12.7,25.4 11.43,26.67 5.08,26.67 B1.+
N$56
  Bottom 0.406: U$2.MASSE 7.39,41.35 U$2.ÖFFNER 7.39,37.05 B1.AC1
N$57  (via drill 0.8 pad 0.81)
  Top 0.305: v42.55,23.81 IC1.7
  Bottom 0.254: JP1.1 29.21,11.43 29.21,13.34 29.84,13.97 31.27,13.97 31.75,13.49 32.86,13.49 33.97,14.61 41.27,14.61 42.55,15.88 IC4.18
  Bottom 0.305: IC4.18 v42.55,23.81

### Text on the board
Top: Drehzahlmesser 1.0 | Top | avr-projekte.de
Bottom: avr-projekte.de | Drehzahlmesser 1.0 | Bottom
Help: D=6mm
